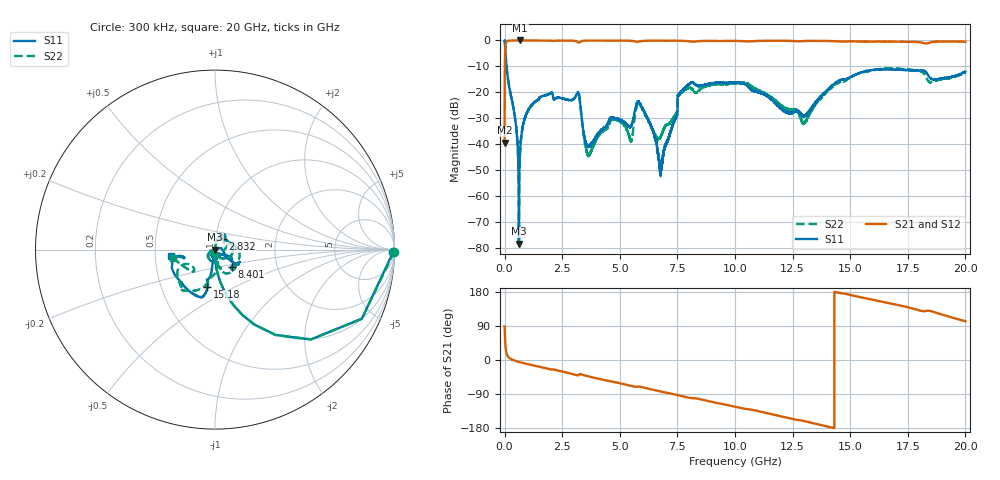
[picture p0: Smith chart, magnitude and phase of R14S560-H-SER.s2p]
!{R14S560}
!Johanson Technology Inc.
!www.johansontechnology.com
!Test Board Conditions:
!Substrate Type  RO4350B
!Substrate Thickness  20 mil
!Substrate Dk  3.66
!TL Type: GCPW
!TL Trace Width  36 mil
!TL Gap  12 mil
!Electrode orientation  Horizontal
!DUT TOPOLOGY	SERIES
!Mounting Pad LxW  26x36 mil
! Created Wed Nov 25 17:33:21 2020
! 2 Port Network Data from SP1.SP block
! freq  magS11  angS11  magS21  angS21  magS12  angS12  magS22  angS22
# khz S ma R 50
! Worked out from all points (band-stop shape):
!   20001 points, 300 kHz to 20 GHz, reference 50 ohm
!   highest |S21| = 0.00 dB at 670.3 MHz (marker M1); lowest = -39.5 dB at 300 kHz (marker M2)
!   |S21| within 3 dB of the highest: 28.45 MHz to end of sweep
!   lowest |S11| = -78.5 dB at 622.3 MHz (marker M3), VSWR 1.00, Z = 50 + j0.00778 ohm
!   |S11| at or under -10 dB: 83.48 MHz to end of sweep
!   |S22| runs from -79.4 to 0.0 dB; largest |S21 - S12| = 0.018
!   S11 on the Smith chart (normalised r, x): 300 kHz: open; 2.832 GHz: 1.08, +0.12; 8.401 GHz: 1.18, -0.23; 15.18 GHz: 0.85, -0.37; 20 GHz: 0.60, -0.05
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300  0.9928 -0.8  0.01062 88.4  0.01057 88.9  0.9976 -0.7
114300  0.2332 -77.4  0.9717 12.5  0.9712 12.5  0.2344 -77.4
622300  0.0001192 40.7  0.9992 -5.0  0.9995 -5.1  0.0003942 -102.8
670300  0.007043 83.1  1 -5.9  0.9992 -5.9  0.006787 84.3
842300  0.02814 81.6  0.9994 -8.6  0.9989 -8.6  0.02733 81.0
1204300  0.05874 75.9  0.9972 -13.7  0.9977 -13.7  0.05835 75.7
2832300  0.07073 53.8  0.9923 -35.2  0.9921 -35.2  0.07042 49.1
3178300  0.09972 6.7  0.9262 -40.8  0.9269 -40.7  0.1006 4.0
3334300  0.03591 -65.6  0.9674 -38.0  0.9681 -38.0  0.03554 -68.9
3662300  0.008834 -80.0  0.9941 -43.7  0.9941 -43.8  0.006219 -120.4
4677300  0.03217 -118.5  0.991 -57.1  0.9914 -57.0  0.02996 -156.0
5480300  0.02206 -92.7  0.9839 -68.3  0.9834 -68.3  0.01174 -126.0
5832300  0.06482 -115.0  0.9547 -70.1  0.9548 -70.1  0.06007 -124.1
6667300  0.006191 170.3  0.9921 -81.6  0.9917 -81.6  0.01255 -103.4
6820300  0.003946 62.5  0.99 -83.7  0.991 -83.7  0.01542 -73.9
7600300  0.09599 -34.0  0.9854 -94.0  0.9859 -93.9  0.09013 18.2
8401300  0.1321 -45.9  0.9675 -102.2  0.9657 -102.2  0.104 3.7
1.00003e7  0.1523 -26.9  0.9778 -123.2  0.9784 -123.2  0.1488 -44.9
1.33343e7  0.05046 -101.4  0.9826 -165.9  0.984 -165.9  0.04524 -72.0
1.51843e7  0.2131 -101.3  0.9601 169.2  0.962 169.0  0.2144 -106.1
1.66673e7  0.2745 -112.0  0.9516 150.2  0.9432 150.1  0.2892 -128.1
2e7  0.2493 -171.2  0.9456 102.2  0.9455 102.4  0.2401 -169.4
